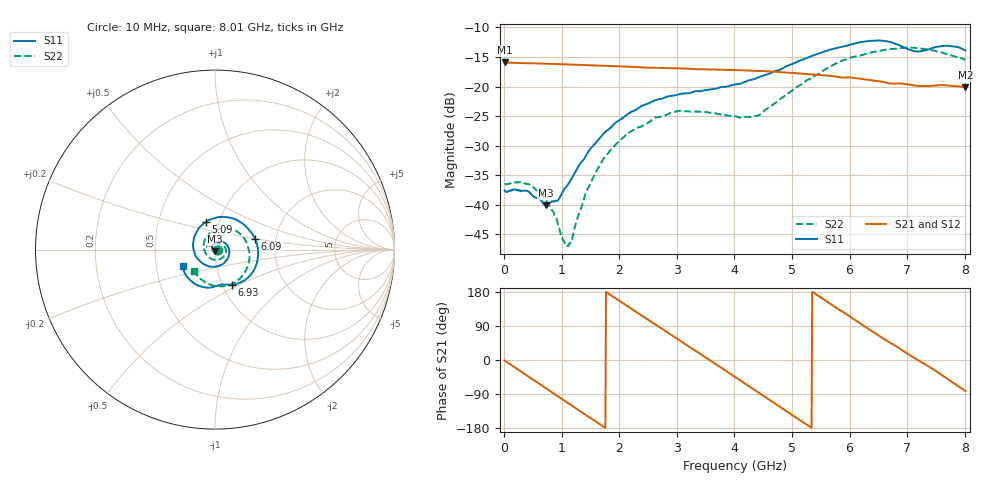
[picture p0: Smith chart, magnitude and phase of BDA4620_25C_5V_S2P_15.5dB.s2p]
!Agilent Technologies,E5071B,MY42404982,A.09.10
!Date: Wed May 06 09:01:30 2026
!Data & Calibration Information:
!Freq	S11:SOLT2(ON)	S21:SOLT2(ON)	S12:SOLT2(ON)	S22:SOLT2(ON)
# Hz S RI R 50
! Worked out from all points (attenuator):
!   801 points, 10 MHz to 8.01 GHz, reference 50 ohm
!   highest |S21| = -15.93 dB at 10 MHz (marker M1); lowest = -20.1 dB at 8.01 GHz (marker M2)
!   lowest |S11| = -40.1 dB at 720 MHz (marker M3), VSWR 1.02, Z = 49.9 - j0.984 ohm
!   |S11| at or under -10 dB: start of sweep to end of sweep
!   |S22| runs from -47.0 to -13.4 dB; largest |S21 - S12| = 0.00065
!   S11 on the Smith chart (normalised r, x): 10 MHz: 1.03, -0.00; 5.09 GHz: 0.86, +0.27; 6.09 GHz: 1.56, +0.19; 6.93 GHz: 1.10, -0.45; 8.01 GHz: 0.69, -0.13
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1e7  0.0132 -0.000872  0.1598 -0.00344  0.1601 -0.0035  0.015 -0.000643
4.4e8  0.00898 -0.00905  0.1104 -0.1122  0.1105 -0.1124  0.0133 -0.00649
7.2e8  -0.000813 -0.00986  0.0428 -0.15  0.0428 -0.1503  0.00697 -0.00875
9.3e8  -0.00913 -0.00582  -0.0146 -0.1542  -0.0148 -0.1543  0.000947 -0.00703
1.09e9  -0.0144 0.000624  -0.057 -0.1431  -0.0571 -0.1432  -0.0035 -0.00285
1.17e9  -0.0156 0.00541  -0.0763 -0.1332  -0.0766 -0.1333  -0.00502 -0.000277
1.35e9  -0.0163 0.0165  -0.1134 -0.1018  -0.1134 -0.1019  -0.00694 0.00688
1.58e9  -0.00958 0.0314  -0.1428 -0.0485  -0.143 -0.0486  -0.00542 0.0175
1.88e9  0.0114 0.045  -0.1461 0.0295  -0.1462 0.0296  0.00518 0.0297
2.68e9  0.0778 0.00392  0.00341 0.1438  0.00359 0.144  0.052 0.0184
3.4e9  0.0349 -0.0844  0.1345 0.0405  0.1347 0.0405  0.0457 -0.0408
4.01e9  -0.0714 -0.0758  0.0982 -0.097  0.0982 -0.0973  -0.0199 -0.0523
4.42e9  -0.1198 -7.71e-05  0.00949 -0.135  0.00937 -0.1352  -0.0564 -0.0108
5.09e9  -0.0529 0.1532  -0.1163 -0.0569  -0.1165 -0.0569  -0.0218 0.0971
5.35e9  0.0208 0.1811  -0.1264 0.000119  -0.1266 0.000243  0.028 0.1155
6.09e9  0.2241 0.0574  -0.0318 0.1137  -0.032 0.114  0.1744 0.0414
6.39e9  0.2364 -0.0608  0.0276 0.1094  0.0277 0.1094  0.1925 -0.0317
6.68e9  0.1747 -0.1641  0.0718 0.0786  0.0722 0.0787  0.1765 -0.1069
6.93e9  0.092 -0.1958  0.0964 0.0429  0.0968 0.0429  0.1369 -0.1632
7.19e9  0.0351 -0.1947  0.1011 -0.000855  0.1014 -0.000879  0.0697 -0.1998
7.58e9  -0.0701 -0.2077  0.0815 -0.0627  0.0817 -0.0627  -0.0361 -0.1916
8.01e9  -0.1797 -0.0924  0.014 -0.0975  0.014 -0.0977  -0.1194 -0.1186
